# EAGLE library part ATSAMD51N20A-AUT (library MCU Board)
120MHZ 1024KB FLASH 100 TQFP PKG Buy Part
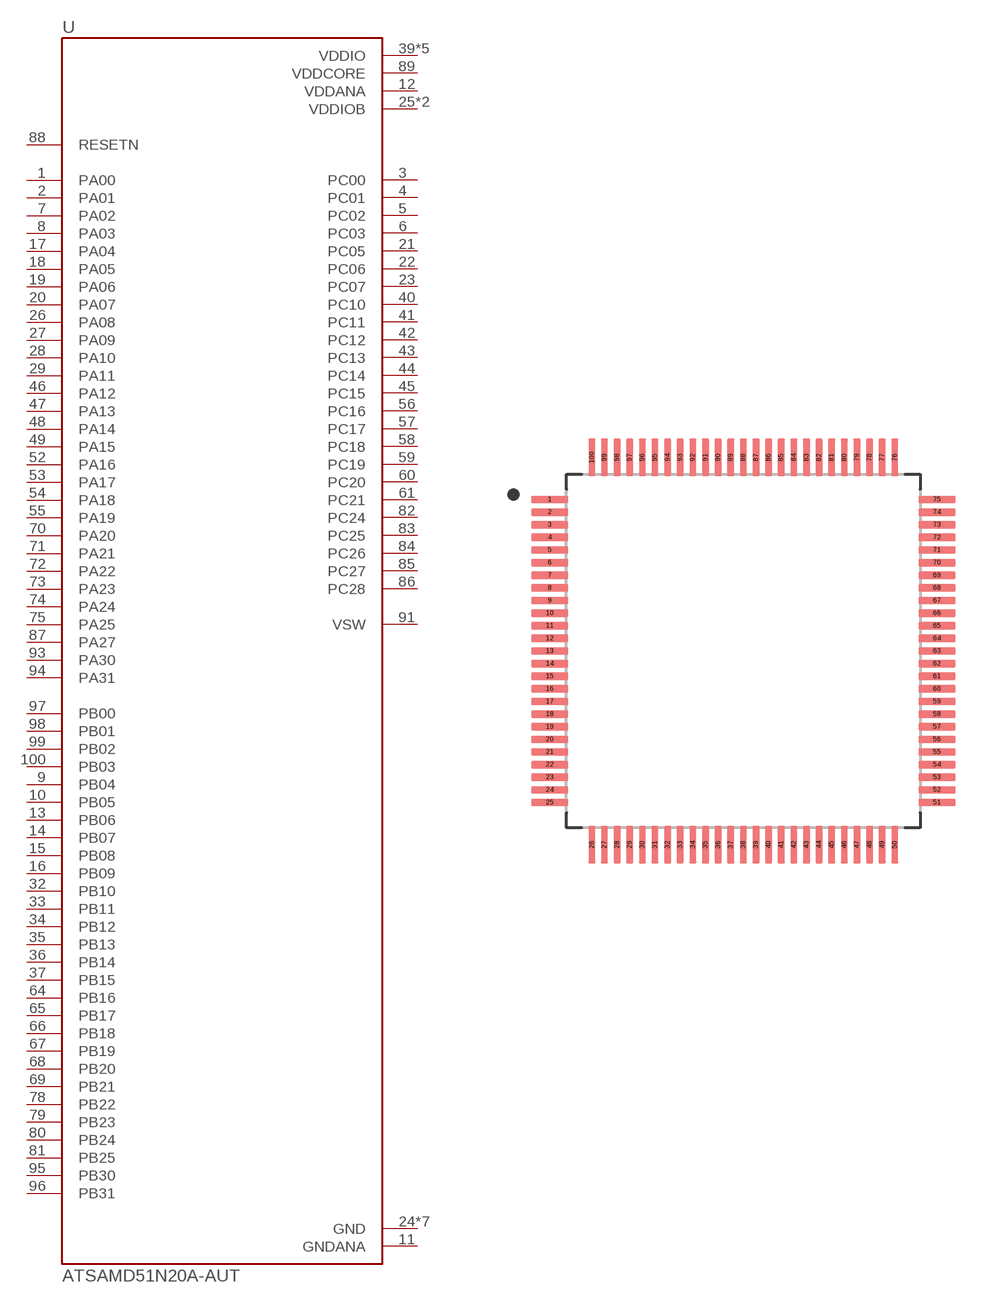
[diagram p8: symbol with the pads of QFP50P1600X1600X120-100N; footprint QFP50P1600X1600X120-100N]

Designator prefix U

## ATSAMD51N20A-AUT (AVAILABILITY: Bad; DESCRIPTION: ARM® Cortex®-M4F SAM D51 Microcontroller IC 32-Bit 120MHz 1MB (1M x 8) FLASH 100-TQFP (14x14); MF: Microchip Technology; MOUSER-PURCHASE-URL: https://snapeda.com/shop?store=Mouser&id=3077901; MP: ATSAMD51N20A-AUT; PACKAGE: TQFP-100 Microchip Technology; PRICE: None)  [QFP50P1600X1600X120-100N]
1  PA00
2  PA01
3  PC00
4  PC01
5  PC02
6  PC03
7  PA02
8  PA03
9  PB04
10  PB05
11  GNDANA  pwr
12  VDDANA  pwr
13  PB06
14  PB07
15  PB08
16  PB09
17  PA04
18  PA05
19  PA06
20  PA07
21  PC05
22  PC06
23  PC07
24  GND  pwr
25  VDDIOB  pwr
26  PA08
27  PA09
28  PA10
29  PA11
30  VDDIOB  pwr
31  GND  pwr
32  PB10
33  PB11
34  PB12
35  PB13
36  PB14
37  PB15
38  GND  pwr
39  VDDIO  pwr
40  PC10
41  PC11
42  PC12
43  PC13
44  PC14
45  PC15
46  PA12
47  PA13
48  PA14
49  PA15
50  GND  pwr
51  VDDIO  pwr
52  PA16
53  PA17
54  PA18
55  PA19
56  PC16
57  PC17
58  PC18
59  PC19
60  PC20
61  PC21
62  GND  pwr
63  VDDIO  pwr
64  PB16
65  PB17
66  PB18
67  PB19
68  PB20
69  PB21
70  PA20
71  PA21
72  PA22
73  PA23
74  PA24
75  PA25
76  GND  pwr
77  VDDIO  pwr
78  PB22
79  PB23
80  PB24
81  PB25
82  PC24
83  PC25
84  PC26
85  PC27
86  PC28
87  PA27
88  RESETN  in
89  VDDCORE  pwr
90  GND  pwr
91  VSW
92  VDDIO  pwr
93  PA30
94  PA31
95  PB30
96  PB31
97  PB00
98  PB01
99  PB02
100  PB03

## Footprint QFP50P1600X1600X120-100N (pad centres in mm)
smd 1.47 x 0.28: 1 -7.67,6; 2 -7.67,5.5; 3 -7.67,5; 4 -7.67,4.5; 5 -7.67,4; 6 -7.67,3.5; 7 -7.67,3; 8 -7.67,2.5; 9 -7.67,2; 10 -7.67,1.5; 11 -7.67,1; 12 -7.67,0.5; 13 -7.67,0; 14 -7.67,-0.5; 15 -7.67,-1; 16 -7.67,-1.5; 17 -7.67,-2; 18 -7.67,-2.5; 19 -7.67,-3; 20 -7.67,-3.5; 21 -7.67,-4; 22 -7.67,-4.5; 23 -7.67,-5; 24 -7.67,-5.5; 25 -7.67,-6; 51 7.67,-6; 52 7.67,-5.5; 53 7.67,-5; 54 7.67,-4.5; 55 7.67,-4; 56 7.67,-3.5; 57 7.67,-3; 58 7.67,-2.5; 59 7.67,-2; 60 7.67,-1.5; 61 7.67,-1; 62 7.67,-0.5; 63 7.67,0; 64 7.67,0.5; 65 7.67,1; 66 7.67,1.5; 67 7.67,2; 68 7.67,2.5; 69 7.67,3; 70 7.67,3.5; 71 7.67,4; 72 7.67,4.5; 73 7.67,5; 74 7.67,5.5; 75 7.67,6
smd 0.28 x 1.47: 26 -6,-7.67; 27 -5.5,-7.67; 28 -5,-7.67; 29 -4.5,-7.67; 30 -4,-7.67; 31 -3.5,-7.67; 32 -3,-7.67; 33 -2.5,-7.67; 34 -2,-7.67; 35 -1.5,-7.67; 36 -1,-7.67; 37 -0.5,-7.67; 38 0,-7.67; 39 0.5,-7.67; 40 1,-7.67; 41 1.5,-7.67; 42 2,-7.67; 43 2.5,-7.67; 44 3,-7.67; 45 3.5,-7.67; 46 4,-7.67; 47 4.5,-7.67; 48 5,-7.67; 49 5.5,-7.67; 50 6,-7.67; 76 6,7.67; 77 5.5,7.67; 78 5,7.67; 79 4.5,7.67; 80 4,7.67; 81 3.5,7.67; 82 3,7.67; 83 2.5,7.67; 84 2,7.67; 85 1.5,7.67; 86 1,7.67; 87 0.5,7.67; 88 0,7.67; 89 -0.5,7.67; 90 -1,7.67; 91 -1.5,7.67; 92 -2,7.67; 93 -2.5,7.67; 94 -3,7.67; 95 -3.5,7.67; 96 -4,7.67; 97 -4.5,7.67; 98 -5,7.67; 99 -5.5,7.67; 100 -6,7.67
